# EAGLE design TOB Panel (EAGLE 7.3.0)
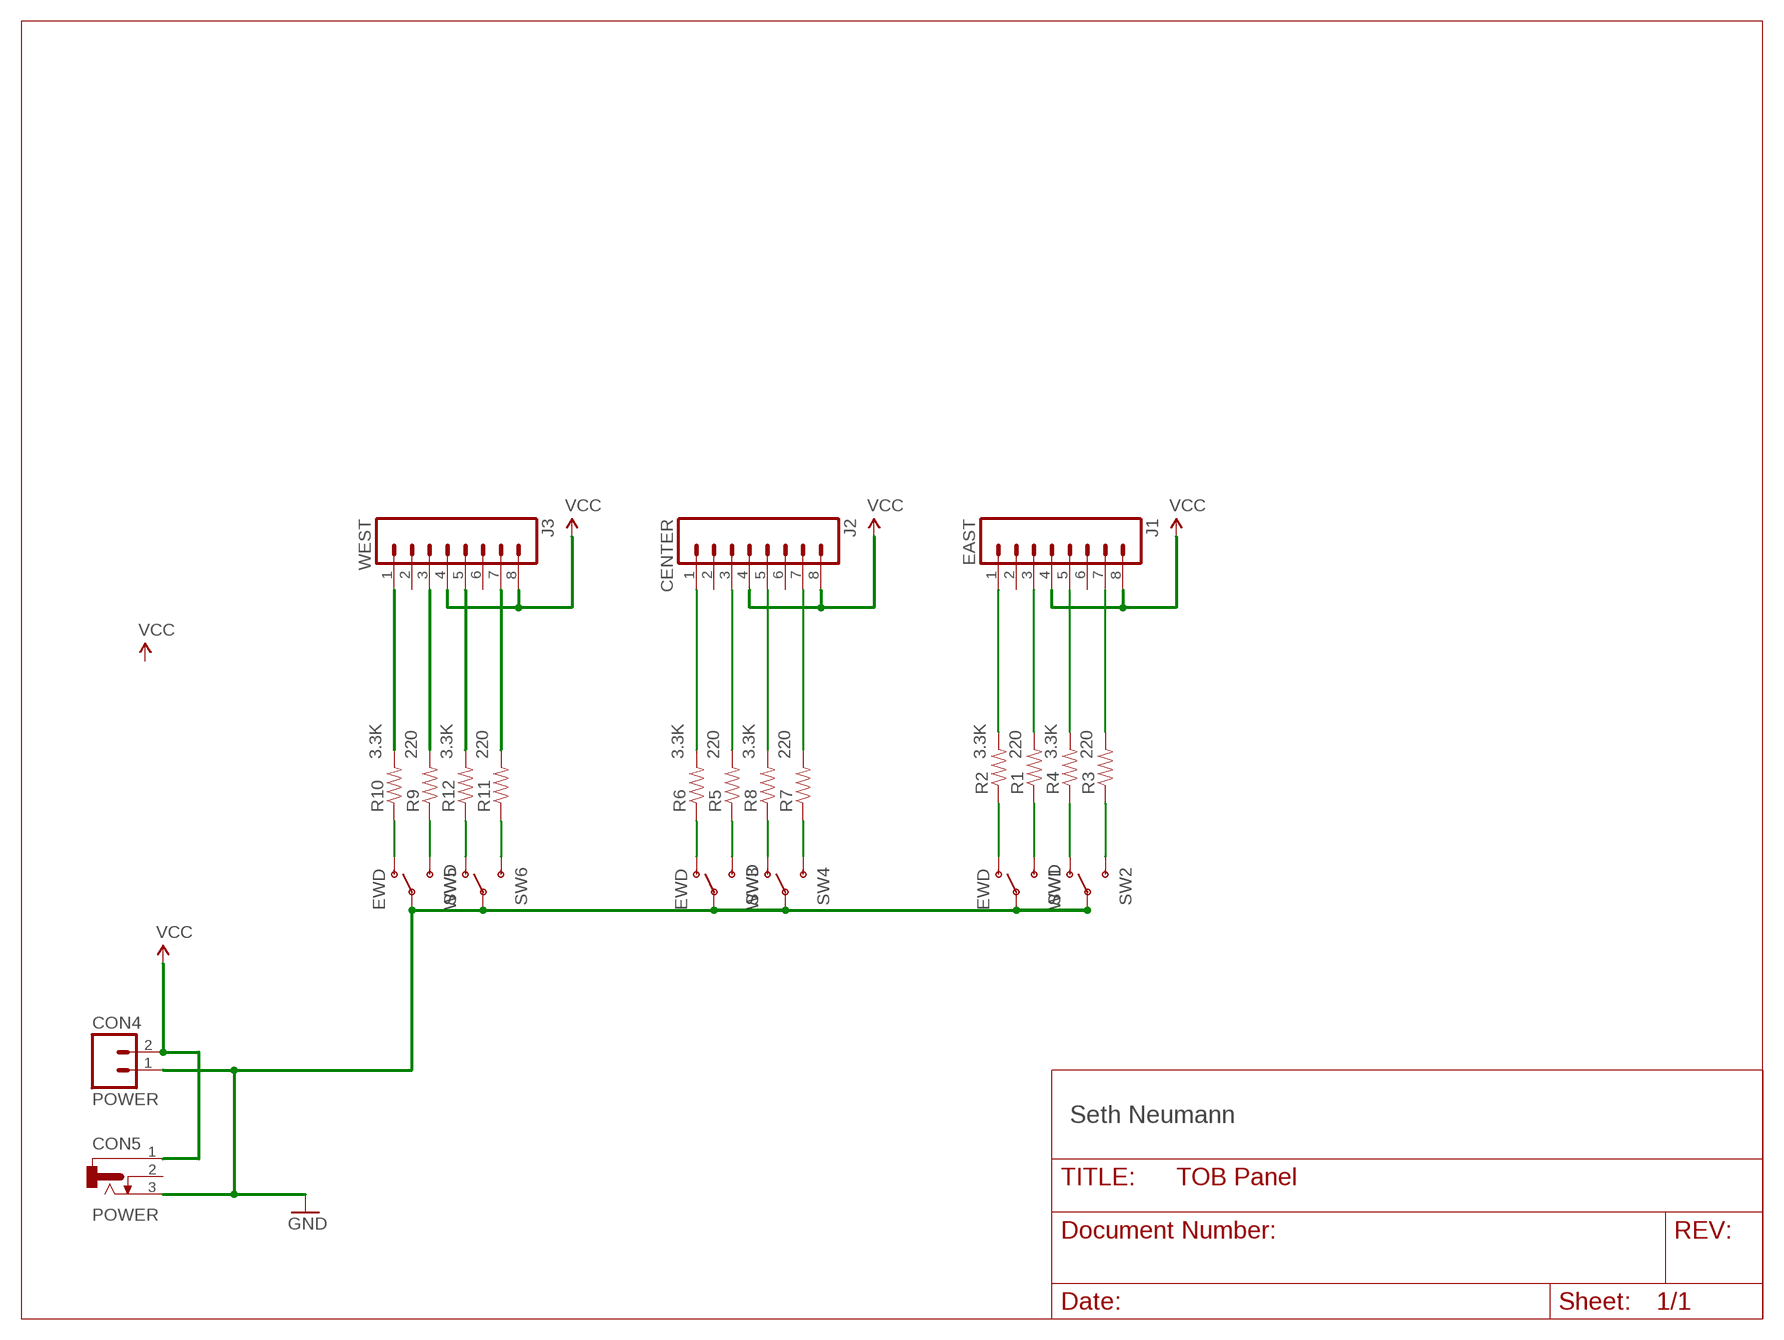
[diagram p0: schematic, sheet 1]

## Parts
CON4  POWER  CONNECTOR-M02MOLEX-1X02-LOCK  [MOLEX-1X2_LOCK]
CON5  POWER  CONNECTOR-DC-POWER-RA  [DCJ0202]
J1  EAST  CONNECTOR-M08FEMALE_LOCK  [1X08_FEMALE_LOCK]
J2  CENTER  CONNECTOR-M08FEMALE_LOCK  [1X08_FEMALE_LOCK]
J3  WEST  CONNECTOR-M08FEMALE_LOCK  [1X08_FEMALE_LOCK]
R1  220  RPTH04  [AXIAL-0.4-RES]
R2  3.3K  RPTH04  [AXIAL-0.4-RES]
R3  220  RPTH04  [AXIAL-0.4-RES]
R4  3.3K  RPTH04  [AXIAL-0.4-RES]
R5  220  RPTH04  [AXIAL-0.4-RES]
R6  3.3K  RPTH04  [AXIAL-0.4-RES]
R7  220  RPTH04  [AXIAL-0.4-RES]
R8  3.3K  RPTH04  [AXIAL-0.4-RES]
R9  220  RPTH04  [AXIAL-0.4-RES]
R10  3.3K  RPTH04  [AXIAL-0.4-RES]
R11  220  RPTH04  [AXIAL-0.4-RES]
R12  3.3K  RPTH04  [AXIAL-0.4-RES]
SW1  EWD  SWITCH-SPSTPTH-508  [SWITCH-SPDT-508]
SW2  WWD  SWITCH-SPSTPTH-508  [SWITCH-SPDT-508]
SW3  EWD  SWITCH-SPSTPTH-508  [SWITCH-SPDT-508]
SW4  WWD  SWITCH-SPSTPTH-508  [SWITCH-SPDT-508]
SW5  EWD  SWITCH-SPSTPTH-508  [SWITCH-SPDT-508]
SW6  WWD  SWITCH-SPSTPTH-508  [SWITCH-SPDT-508]

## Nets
GND: CON4.1(A) CON5.3 SW1.2(P) SW2.2(P) SW3.2(P) SW4.2(P) SW5.2(P) SW6.2(P)
N$1: J1.3 R1.P$2
N$2: R4.P$1 SW2.1(O)
N$3: J1.1 R2.P$2
N$4: R3.P$1 SW2.3(S)
N$5: J1.7 R3.P$2
N$6: J1.5 R4.P$2
N$7: R2.P$1 SW1.1(O)
N$8: R1.P$1 SW1.3(S)
N$9: J2.7 R7.P$2
N$10: J2.5 R8.P$2
N$11: J2.3 R5.P$2
N$12: J2.1 R6.P$2
N$13: R8.P$1 SW4.1(O)
N$14: R7.P$1 SW4.3(S)
N$15: R6.P$1 SW3.1(O)
N$16: R5.P$1 SW3.3(S)
N$17: R9.P$1 SW5.3(S)
N$18: R10.P$1 SW5.1(O)
N$19: R11.P$1 SW6.3(S)
N$20: R12.P$1 SW6.1(O)
N$21: J3.1 R10.P$2
N$22: J3.3 R9.P$2
N$23: J3.5 R12.P$2
N$24: J3.7 R11.P$2
VCC: CON4.2(B) CON5.1 J1.4 J1.8 J2.4 J2.8 J3.4 J3.8
Unconnected: CON5.2 J1.2 J1.6 J2.2 J2.6 J3.2 J3.6

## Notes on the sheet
- Seth Neumann

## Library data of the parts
CON4 = SPCoast:CONNECTOR-M02: PHOENIX CONNECTOR
CON5 = SPCoast:CONNECTOR-DC-POWER: DC POWER JACK
J1-J3 = SPCoast:CONNECTOR-M08: Header 8 Standard 8-pin 0.1" header. Use with straight break away headers (SKU : PRT-00116), right angle break away headers (PRT-00553), swiss pins (PRT-00743), machine pins (PRT-00117), and female headers (PRT-00115).
R1-R12 = SPCoast:R*: Resistor
SW1-SW6 = SPCoast:SWITCH-SPST: SPST Switch Simple slide switch. Spark Fun Electronics SKU : COM-00102

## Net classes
0 default: width 0.254 mm, clearance 0.254 mm
1 Power: width 0.406 mm, clearance 0.254 mm
2 Phone: width 0.305 mm, clearance 0.381 mm
3 Nasty Loads: width 0.61 mm, clearance 0.61 mm

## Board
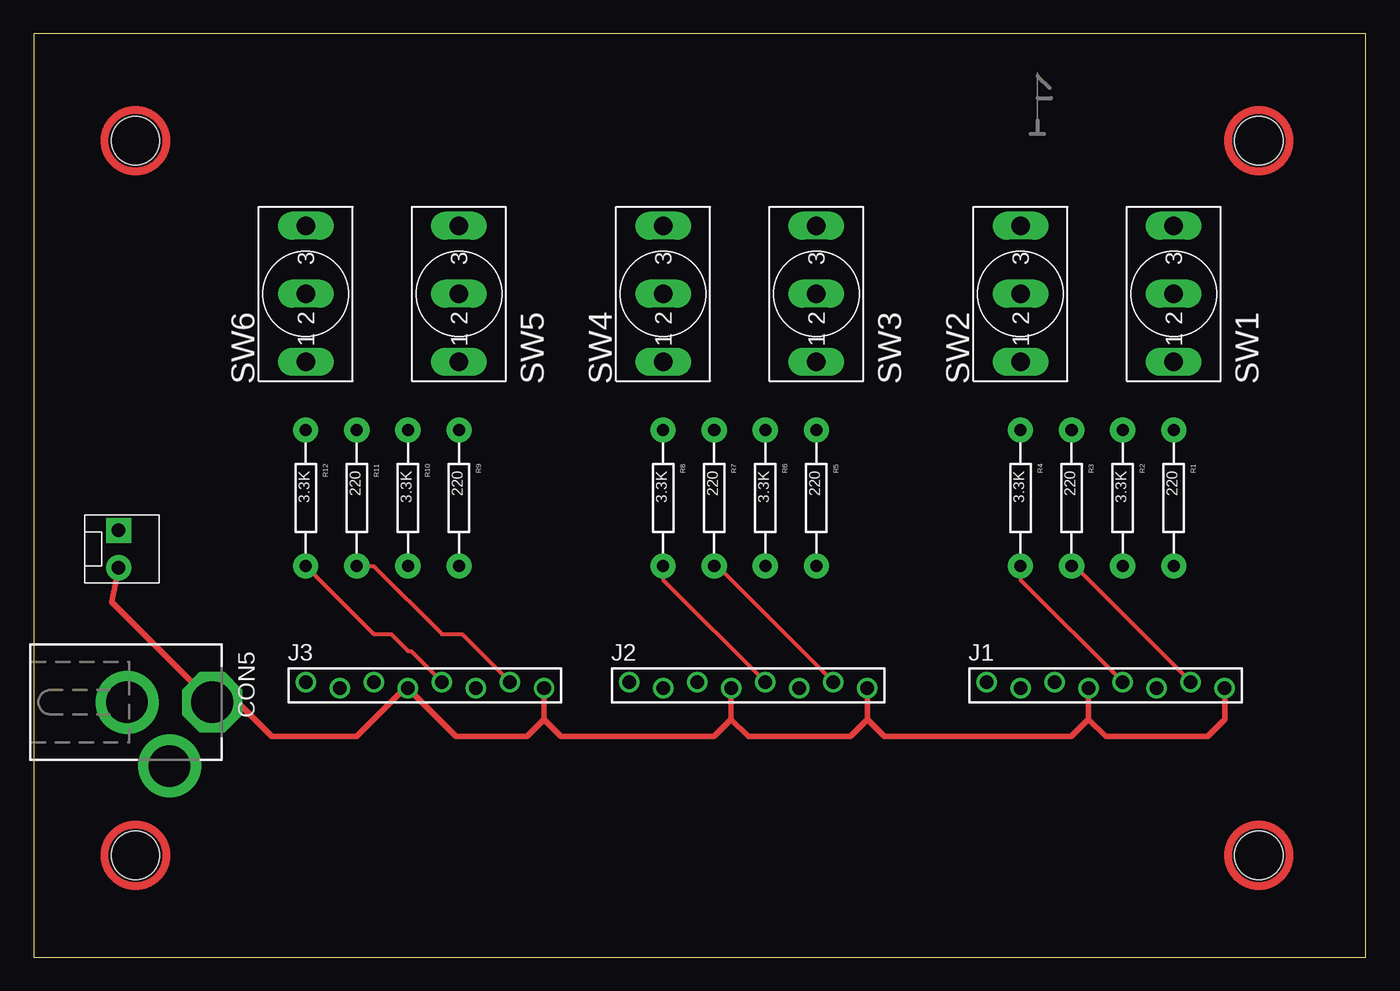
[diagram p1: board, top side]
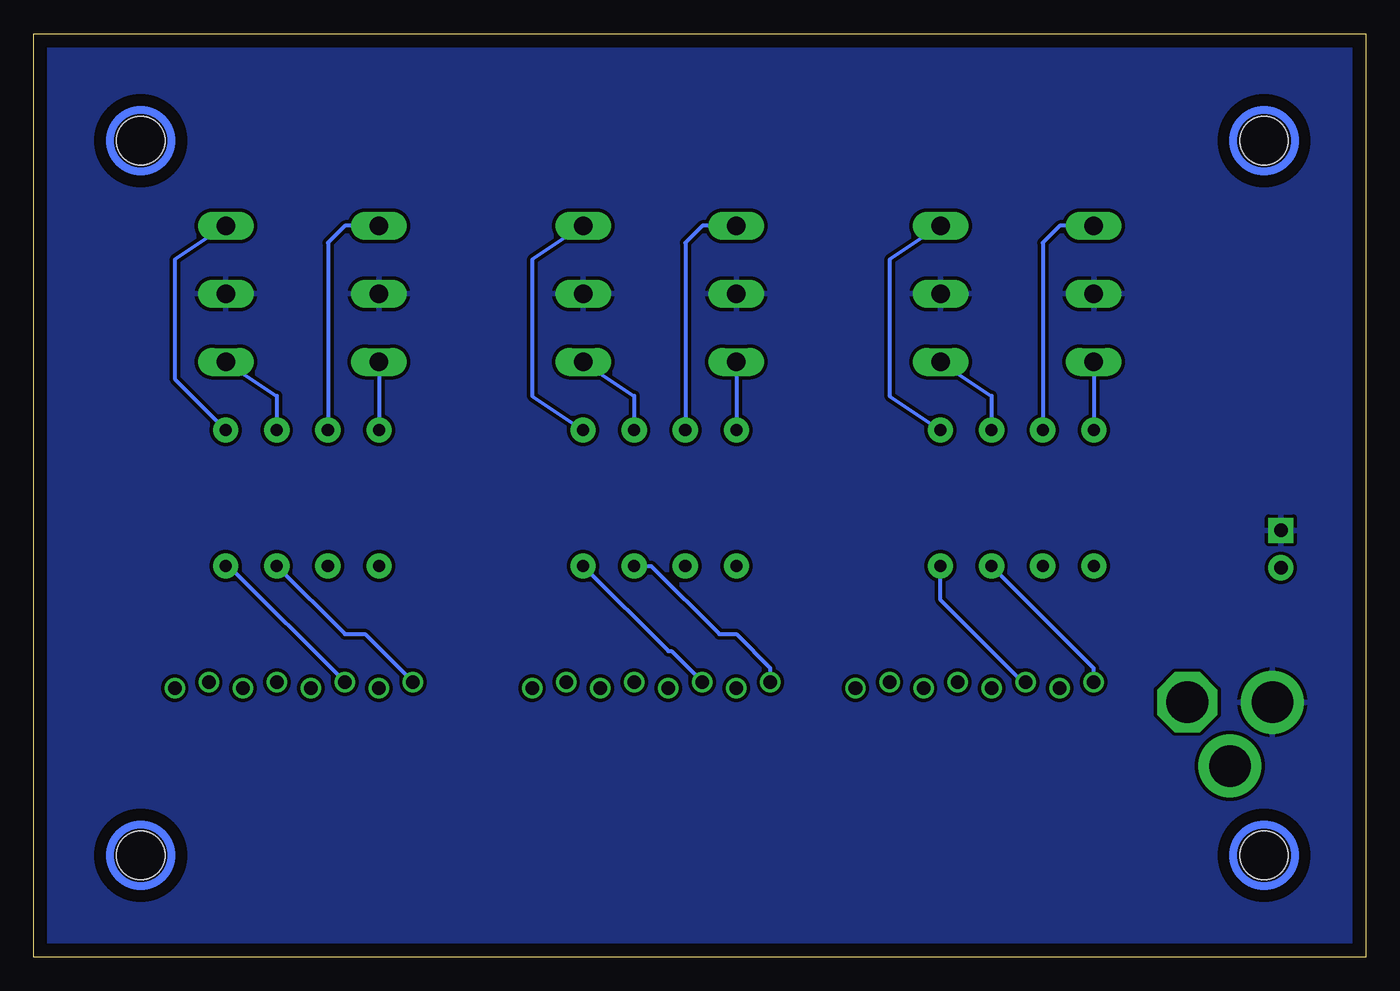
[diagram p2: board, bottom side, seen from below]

Size 99.44 x 68.96 mm. Coordinates in mm from the lower left corner, seen from the top.
Outline: 0,0 99.44,0 99.44,68.96 0,68.96 0,0
Copper layers (1*16): Top 0.035mm / dielectric 1.5mm / Bottom 0.035mm
Design rules "default": minimum track width 10mil, minimum drill 0.6mm, track to track 8mil, track to pad 8mil, pad to pad 8mil, via to via 8mil, smd to smd 8mil, copper to edge 40mil, drill to drill 8mil, minimum pad ring 10mil, minimum via ring 8mil, stop-mask expansion 4mil, vias tented up to drill 0mil, thermal gap 10mil

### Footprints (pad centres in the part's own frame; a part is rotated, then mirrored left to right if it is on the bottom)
MOLEX-1X2_LOCK = drill 1.016 pad 1.88 square: 1 -0.127,0 | drill 1.016 pad 1.88: 2 2.667,0
DCJ0202 = drill 3.1 pad 4.5 octagon: 1 0,3.175 | drill 3.1 pad 4.7: 2 4.763,0; 3 0,-3.175
1X08_FEMALE_LOCK = drill 1.016: 1 0,0.229; 2 2.54,-0.229; 3 5.08,0.229; 4 7.62,-0.229; 5 10.16,0.229; 6 12.7,-0.229; 7 15.24,0.229; 8 17.78,-0.229
AXIAL-0.4-RES = drill 0.9 pad 1.88: P$1 -5.08,0; P$2 5.08,0
SWITCH-SPDT-508 = drill 1.397 long: 1 -5.08,0; 2 0,0; 3 5.08,0
MOUNTINGHOLE = hole 3.6: 0,0

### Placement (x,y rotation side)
CON4  6.35,31.75 270 top
CON5  10.16,19.05 270 top
J1  71.12,20.32 0 top
J2  44.45,20.32 0 top
J3  20.32,20.32 0 top
R1  85.09,34.29 270 top
R2  81.28,34.29 270 top
R3  77.47,34.29 270 top
R4  73.66,34.29 270 top
R5  58.42,34.29 270 top
R6  54.61,34.29 270 top
R7  50.8,34.29 270 top
R8  46.99,34.29 270 top
R9  31.75,34.29 270 top
R10  27.94,34.29 270 top
R11  24.13,34.29 270 top
R12  20.32,34.29 270 top
SW1  85.09,49.53 90 top
SW2  73.66,49.53 90 top
SW3  58.42,49.53 90 top
SW4  46.99,49.53 90 top
SW5  31.75,49.53 90 top
SW6  20.32,49.53 90 top
U$1  [MOUNTINGHOLE]  7.62,60.96 0 top
U$2  [MOUNTINGHOLE]  91.44,60.96 0 top
U$3  [MOUNTINGHOLE]  91.44,7.62 0 top
U$4  [MOUNTINGHOLE]  7.62,7.62 0 top
U$5  [MRCSLOGOTOP]  73.66,60.96 0 top
U$6  [CA-PROP65WARNING]  36.83,35.56 0 top

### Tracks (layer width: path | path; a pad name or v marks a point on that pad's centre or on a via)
GND
  pour Bottom (isolate 0): 0,0 0,68.58 99.06,68.58 99.06,0
N$1
  Bottom 0.305: R1.P$2 84.86,29.21 J1.3
N$2
  Bottom 0.305: SW2.1 R4.P$1
N$3
  Bottom 0.305: R2.P$2 76.2,24.13 74.7,24.13 J1.1
N$4
  Bottom 0.305: SW2.3 76.2,54.61 77.47,53.34 R3.P$1
N$5
  Top 0.305: R3.P$2 77.7,29.21 J1.7
N$6
  Top 0.305: R4.P$2 73.66,28.17 J1.5
N$7
  Bottom 0.305: SW1.1 81.28,41.91 R2.P$1
N$8
  Bottom 0.305: SW1.3 88.9,52.07 88.9,43.18 R1.P$1
N$9
  Top 0.305: R7.P$2 51.03,29.21 J2.7
N$10
  Top 0.305: R8.P$2 46.99,28.17 J2.5
N$11
  Bottom 0.305: R5.P$2 52.07,22.86 51.84,22.86 J2.3
N$12
  Bottom 0.305: J2.1 44.45,21.59 46.99,24.13 48.26,24.13 53.34,29.21 R6.P$2
N$13
  Bottom 0.305: SW4.1 R8.P$1
N$14
  Bottom 0.305: SW4.3 49.53,54.61 50.8,53.34 R7.P$1
N$15
  Bottom 0.305: SW3.1 54.61,41.91 R6.P$1
N$16
  Bottom 0.305: SW3.3 62.23,52.07 62.23,41.91 R5.P$1
N$17
  Bottom 0.305: SW5.3 35.56,52.07 35.56,41.91 R9.P$1
N$18
  Bottom 0.305: SW5.1 27.94,41.91 R10.P$1
N$19
  Bottom 0.305: SW6.3 22.86,54.61 24.13,53.34 R11.P$1
N$20
  Bottom 0.305: SW6.1 R12.P$1
N$21
  Bottom 0.305: J3.1 20.32,21.59 R10.P$2
N$22
  Bottom 0.305: J3.3 25.63,20.55 31.75,26.67 R9.P$2
N$23
  Top 0.305: R12.P$2 25.4,24.13 26.67,24.13 27.94,22.86 28.17,22.86 J3.5
N$24
  Top 0.305: R11.P$2 25.4,29.21 30.48,24.13 31.98,24.13 J3.7
VCC
  Top 0.406: CON4.2 5.84,26.54 CON5.1 15.24,19.05 17.78,16.51 24.13,16.51 27.71,20.09 J3.4 31.52,16.51 36.83,16.51 38.1,17.78 | J3.8 38.1,17.78 | 38.1,17.78 39.37,16.51 50.8,16.51 52.07,17.78 | J2.4 52.07,17.78 | 52.07,17.78 53.34,16.51 60.96,16.51 62.23,17.78 | J2.8 62.23,17.78 | 62.23,17.78 63.5,16.51 77.47,16.51 78.74,17.78 | J1.4 78.74,17.78 | 78.74,17.78 80.01,16.51 87.63,16.51 88.9,17.78 J1.8

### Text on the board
tDocu: 3 x TOB Switch Panel / 20200216 / Seth Neumann | GND / +V | WH/BL CLR / BL/WH / WH/OR STP / OR/WH +V / WH/GN CLR / GN/WH / WH/BN STP / BN/WH +V | WH/BL CLR / BL/WH / WH/OR STP / OR/WH +V / WH/GN CLR / GN/WH / WH/BN STP / BN/WH +V | WH/BL CLR / BL/WH / WH/OR STP / OR/WH +V / WH/GN CLR / GN/WH / WH/BN STP / BN/WH +V
bDocu: WEST SWITCHES ON THIS SIDE EAST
